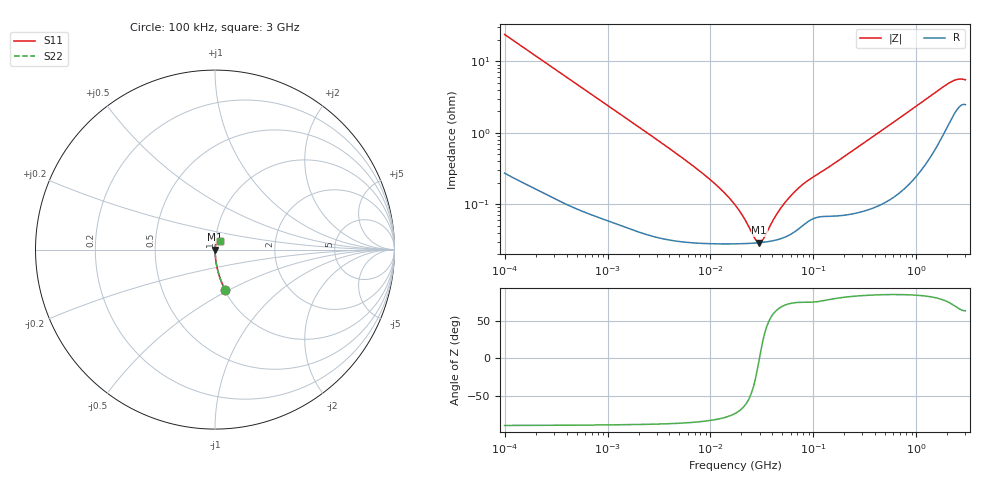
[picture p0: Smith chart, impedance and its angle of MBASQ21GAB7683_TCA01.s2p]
! MBASQ21GAB7683_TCA01  S-PARAMETER MODEL  ( Standard Model )
! Model Generated by TAIYO YUDEN Corporation (http://www.ty-top.com)
! Version 1.0
! TAIYO YUDEN Control No. 220901
! Copyright(c) 2022 TAIYO YUDEN CO.,LTD. All Rights Reserved.
! Product Description (link to TY-COMPAS)
! https://ds.yuden.co.jp/TYCOMPAS/or/detail?pn=MBASQ21GAB7683KTCA01&u=M
! Products Name : Multilayer Ceramic Capacitors
! Characteristics :
!  Capacitance : 0.068 [uF] , Rated Voltage : 250 [V] , TCC : X7R
!  Case Size : 2.0 x 1.25 / 0.079 x 0.049 [mm/inch] , Thickness : 1.25 / 0.049 [mm/inch]
!  (Conditions: Temperature = 25 [degC] , DC Bias Voltage = 0 [V])
! External Node Assignments :
!  1  o---| |---o  2
! GND o---------o GND
! Frequency Range : 100kHz  -  3GHz  [ 401 STEP ]
# MHZ S RI R 50
! Freq[MHz].  S11 Real  S11 Imag  S21 Real  S21 Imag  S12 Real  S12 Imag  S22 Real  S22 Imag
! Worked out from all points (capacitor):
!   401 points, 100 kHz to 3 GHz, reference 50 ohm
!   read as one part in series: C = 67.1 nF near 105.3 kHz
!   lowest |Z| = 29 mohm at 29.76 MHz (marker M1)
!   series resonance near 29.93 MHz, so ESL is about 420 pH
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0.1  0.0554 -0.223  0.9446 0.223  0.9446 0.223  0.0554 -0.223
0.222319  0.0128 -0.1055  0.9872 0.1055  0.9872 0.1055  0.0128 -0.1055
0.562235  0.00261 -0.0425  0.9974 0.0425  0.9974 0.0425  0.00261 -0.0425
3.161081  0.000396 -0.00762  0.9996 0.00762  0.9996 0.00762  0.000396 -0.00762
6.178009  0.000305 -0.00378  0.9997 0.00378  0.9997 0.00378  0.000305 -0.00378
9.824692  0.000285 -0.00222  0.9997 0.00222  0.9997 0.00222  0.000285 -0.00222
13.7349  0.00028 -0.00141  0.9997 0.00141  0.9997 0.00141  0.00028 -0.00141
17.7727  0.00028 -0.000892  0.9997 0.000892  0.9997 0.000892  0.00028 -0.000892
21.28644  0.000281 -0.000569  0.9997 0.000569  0.9997 0.000569  0.000281 -0.000569
26.84345  0.000286 -0.000179  0.9997 0.000179  0.9997 0.000179  0.000286 -0.000179
28.26337  0.000288 -9.38e-05  0.9997 9.38e-05  0.9997 9.38e-05  0.000288 -9.38e-05
29.75839  0.000289 -9.16e-06  0.9997 9.16e-06  0.9997 9.16e-06  0.000289 -9.16e-06
31.3325  0.000292 7.55e-05  0.9997 -7.55e-05  0.9997 -7.55e-05  0.000292 7.55e-05
32.98988  0.000294 0.00016  0.9997 -0.00016  0.9997 -0.00016  0.000294 0.00016
42.68829  0.000314 0.000598  0.9997 -0.000598  0.9997 -0.000598  0.000314 0.000598
53.83243  0.000351 0.00103  0.9996 -0.00103  0.9996 -0.00103  0.000351 0.00103
71.47675  0.000451 0.00161  0.9995 -0.00161  0.9995 -0.00161  0.000451 0.00161
97.38194  0.000622 0.00227  0.9994 -0.00227  0.9994 -0.00227  0.000622 0.00227
547.5153  0.0013 0.0127  0.9987 -0.0127  0.9987 -0.0127  0.0013 0.0127
2038.117  0.0146 0.0457  0.9854 -0.0457  0.9854 -0.0457  0.0146 0.0457
2504.792  0.0234 0.0492  0.9766 -0.0492  0.9766 -0.0492  0.0234 0.0492
3000  0.0264 0.0468  0.9736 -0.0468  0.9736 -0.0468  0.0264 0.0468
